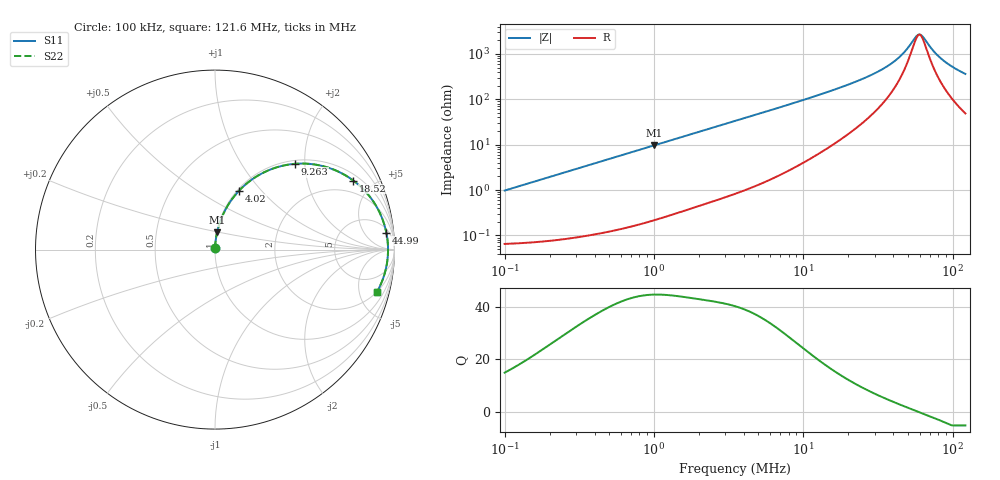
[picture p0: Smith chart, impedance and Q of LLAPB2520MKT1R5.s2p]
! LLAPB2520MKT1R5  S-PARAMETER MODEL  ( General Type )
! Model Generated by TAIYO YUDEN Corporation (http://www.ty-top.com)
! Version 1.0
! TAIYO YUDEN Control No. 151211NG33SB-FKC
! Copyright(c) 2015 TAIYO YUDEN CO.,LTD. All Rights Reserved.
! Product Description (link to TY-COMPAS)
! https://ds.yuden.co.jp/TYCOMPAS/or/detail?pn=LLAPB2520MKT1R5M&u=M
! Products Name : Inductors
! Characteristics :
!  Inductance : 1.5 uH , SRF(min) : -Hz , DC Resistance(max) : 0.065 Ohm
!  Rated Current : Saturation :3300 mA , Temp Rise : 2600 mA (40 degC)
!  Case Size : 2.5 x 2.0 / 0.098 x 0.079 [mm/inch] , Thickness : 1.2 / 0.047 [mm/inch]
!  (Conditions: Temperature = 25 degC , DC Bias Current/Voltage = 0A / 0V)
! External Node Assignments :
!  1  o---GGG---o  2
! GND o---------o GND
! Frequency Range : 0.1MHz  -  121.638923MHz  [ 402 STEP ]
# MHz S RI R 50
! Freq[MHz].  S11 Real  S11 Imag  S21 Real  S21 Imag  S12 Real  S12 Imag  S22 Real  S22 Imag
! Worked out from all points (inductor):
!   401 points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, 100 kHz to 121.6 MHz, reference 50 ohm
!   read as one part in series: L = 1.55 uH near 103.6 kHz
!   highest Q = 44.5 at 1.006 MHz (marker M1), where L = 1.53 uH
!   self-resonance near 59.86 MHz
!   S11 on the Smith chart (normalised r, x): 100 kHz: 1.00, +0.02; 4.02 MHz: 1.02, +0.76; 9.263 MHz: 1.07, +1.79; 18.52 MHz: 1.29, +3.84; 44.99 MHz: 7, +17; 121.6 MHz: 1.98, -7.19
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0.1  0.000745 0.00972  0.9993 -0.00972  0.9993 -0.00972  0.000745 0.00972
0.328662  0.00195 0.0317  0.998 -0.0317  0.998 -0.0317  0.00195 0.0317
1.006117  0.0113 0.0953  0.9887 -0.0953  0.9887 -0.0953  0.0113 0.0953
1.080188  0.0129 0.1021  0.9871 -0.1021  0.9871 -0.1021  0.0129 0.1021
2.159205  0.0448 0.1955  0.9552 -0.1955  0.9552 -0.1955  0.0448 0.1955
3.550168  0.1081 0.2983  0.8919 -0.2983  0.8919 -0.2983  0.1081 0.2983
4.020108  0.1336 0.3276  0.8664 -0.3276  0.8664 -0.3276  0.1336 0.3276
6.048245  0.2558 0.4217  0.7442 -0.4217  0.7442 -0.4217  0.2558 0.4217
9.262618  0.4463 0.478  0.5537 -0.478  0.5537 -0.478  0.4463 0.478
11.46267  0.5541 0.4744  0.4459 -0.4744  0.4459 -0.4744  0.5541 0.4744
18.5152  0.7707 0.3847  0.2293 -0.3847  0.2293 -0.3847  0.7707 0.3847
27.85608  0.89 0.256  0.11 -0.256  0.11 -0.256  0.89 0.256
37.67347  0.9387 0.154  0.0613 -0.154  0.0613 -0.154  0.9387 0.154
44.99481  0.9547 0.0945  0.0453 -0.0945  0.0453 -0.0945  0.9547 0.0945
49.1729  0.9597 0.065  0.0403 -0.065  0.0403 -0.065  0.9597 0.065
56.67966  0.9638 0.018  0.0362 -0.018  0.0362 -0.018  0.9638 0.018
60.85244  0.9641 -0.00543  0.0359 0.00543  0.0359 0.00543  0.9641 -0.00543
64.18241  0.9636 -0.023  0.0364 0.023  0.0364 0.023  0.9636 -0.023
75.3061  0.9582 -0.0759  0.0418 0.0759  0.0418 0.0759  0.9582 -0.0759
83.77342  0.9512 -0.1114  0.0488 0.1114  0.0488 0.1114  0.9512 -0.1114
100.0537  0.9328 -0.1712  0.0672 0.1712  0.0672 0.1712  0.9328 -0.1712
121.6389  0.9017 -0.2375  0.0983 0.2375  0.0983 0.2375  0.9017 -0.2375
